FUNCTION FC 85 : VOID
TITLE =BLOCK FOR START SLIDE ADJUSTMENT
AUTHOR : Esposito
FAMILY : EGAL_srl
NAME : SLIDE_AD
VERSION : 0.1

BEGIN
NETWORK
TITLE =CONDITIONS FOR START SLIDE ADJUSTMENT
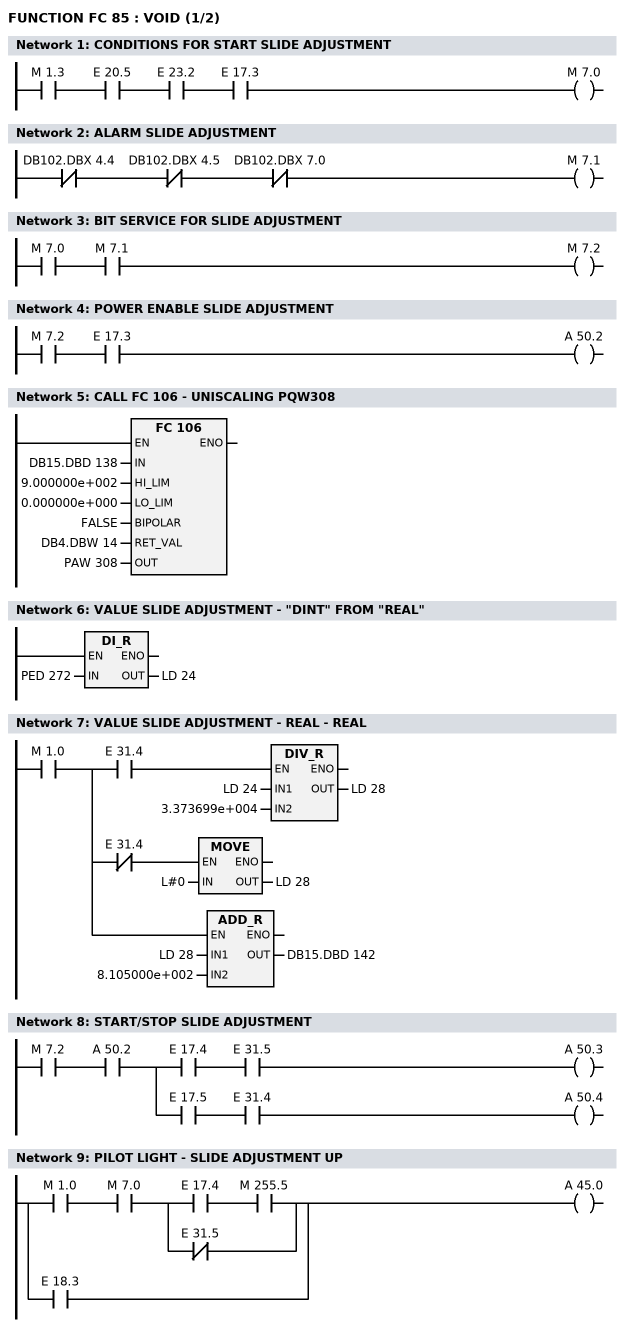
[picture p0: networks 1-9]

      U     M      1.3;
      U     E     20.5;
      U     E     23.2;
      U     E     17.3;
      =     M      7.0;
NETWORK
TITLE =ALARM SLIDE ADJUSTMENT

      UN    DB102.DBX    4.4;
      UN    DB102.DBX    4.5;
      UN    DB102.DBX    7.0;
      =     M      7.1;
NETWORK
TITLE =BIT SERVICE FOR SLIDE ADJUSTMENT

      U     M      7.0;
      U     M      7.1;
      =     M      7.2;
NETWORK
TITLE =POWER ENABLE SLIDE ADJUSTMENT

      U     M      7.2;
      U     E     17.3;
      =     A     50.2;
NETWORK
TITLE =CALL FC 106 - UNISCALING PQW308

      CALL FC   106 (
           IN                       := DB15.DBD  138,
           HI_LIM                   := 9.000000e+002,
           LO_LIM                   := 0.000000e+000,
           BIPOLAR                  := FALSE,
           RET_VAL                  := DB4.DBW   14,
           OUT                      := PAW  308);

NETWORK
TITLE =VALUE SLIDE ADJUSTMENT - "DINT" FROM "REAL"

      L     PED  272;
      DTR   ;
      T     LD    24;
NETWORK
TITLE =VALUE SLIDE ADJUSTMENT - REAL - REAL



      U     M      1.0;
      =     L     32.0;
      U     L     32.0;
      U     E     31.4;
      SPBNB _001;
      L     LD    24;
      L     3.373699e+004;
      /R    ;
      T     LD    28;
_001: NOP   0;
      U     L     32.0;
      UN    E     31.4;
      SPBNB _002;
      L     L#0;
      T     LD    28;
_002: NOP   0;
      U     L     32.0;
      SPBNB _003;
      L     LD    28;
      L     8.105000e+002;
      +R    ;
      T     DB15.DBD  142;
_003: NOP   0;
NETWORK
TITLE =START/STOP SLIDE ADJUSTMENT

      U     M      7.2;
      U     A     50.2;
      =     L     32.0;
      U     L     32.0;
      U     E     17.4;
      U     E     31.5;
      =     A     50.3;
      U     L     32.0;
      U     E     17.5;
      U     E     31.4;
      =     A     50.4;
NETWORK
TITLE =PILOT LIGHT - SLIDE ADJUSTMENT UP

      U     M      1.0;
      U     M      7.0;
      U(    ;
      U     E     17.4;
      U     M    255.5;
      ON    E     31.5;
      )     ;
      O     E     18.3;
      =     A     45.0;
NETWORK
TITLE =PILOT LIGHT - SLIDE ADJUSTMENT DOWN
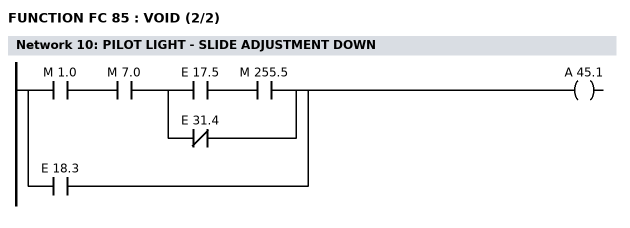
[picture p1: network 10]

      U     M      1.0;
      U     M      7.0;
      U(    ;
      U     E     17.5;
      U     M    255.5;
      ON    E     31.4;
      )     ;
      O     E     18.3;
      =     A     45.1;
END_FUNCTION

